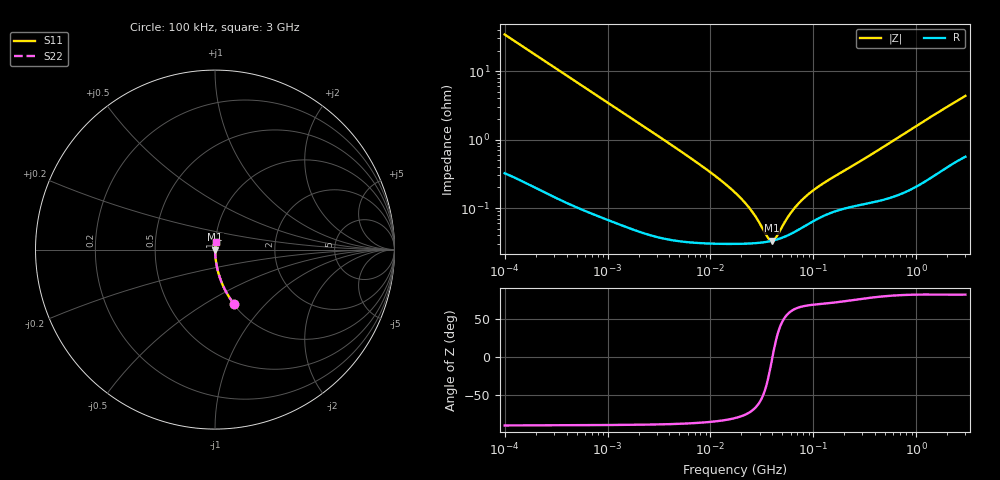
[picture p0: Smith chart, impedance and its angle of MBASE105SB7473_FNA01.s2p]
! MBASE105SB7473_FNA01  S-PARAMETER MODEL  ( Standard Model )
! Model Generated by TAIYO YUDEN Corporation (http://www.ty-top.com)
! Version 1.0
! TAIYO YUDEN Control No. 220601
! Copyright(c) 2013 TAIYO YUDEN CO.,LTD. All Rights Reserved.
! Product Description (link to TY-COMPAS)
! https://ds.yuden.co.jp/TYCOMPAS/or/detail?pn=MBASE105SB7473KFNA01&u=M
! Products Name : Multilayer Ceramic Capacitors
! Characteristics :
!  Capacitance : 0.047 [uF] , Rated Voltage : 16 [V] , TCC : X7R
!  Case Size : 1.0 x 0.5 / 0.039 x 0.02 [mm/inch] , Thickness : 0.5 / 0.02 [mm/inch]
!  (Conditions: Temperature = 25 [degC] , DC Bias Voltage = 0 [V])
! External Node Assignments :
!  1  o---| |---o  2
! GND o---------o GND
! Frequency Range : 100kHz  -  3GHz  [ 401 STEP ]
# MHZ S RI R 50
! Freq[MHz].  S11 Real  S11 Imag  S21 Real  S21 Imag  S12 Real  S12 Imag  S22 Real  S22 Imag
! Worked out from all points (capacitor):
!   401 points, 100 kHz to 3 GHz, reference 50 ohm
!   read as one part in series: C = 46.3 nF near 105.3 kHz
!   lowest |Z| = 33.3 mohm at 39.51 MHz (marker M1)
!   series resonance near 39.99 MHz, so ESL is about 340 pH
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0.1  0.1078 -0.3054  0.8922 0.3054  0.8922 0.3054  0.1078 -0.3054
0.147195  0.054 -0.2208  0.946 0.2208  0.946 0.2208  0.054 -0.2208
0.228123  0.0241 -0.1475  0.9759 0.1475  0.9759 0.1475  0.0241 -0.1475
0.562235  0.00474 -0.0614  0.9953 0.0614  0.9953 0.0614  0.00474 -0.0614
3.161081  0.000493 -0.0111  0.9995 0.0111  0.9995 0.0111  0.000493 -0.0111
9.574722  0.000316 -0.00348  0.9997 0.00348  0.9997 0.00348  0.000316 -0.00348
17.7727  0.000302 -0.0016  0.9997 0.0016  0.9997 0.0016  0.000302 -0.0016
24.21403  0.000304 -0.000929  0.9997 0.000929  0.9997 0.000929  0.000304 -0.000929
28.26337  0.000309 -0.000629  0.9997 0.000629  0.9997 0.000629  0.000309 -0.000629
35.64176  0.000322 -0.000205  0.9997 0.000205  0.9997 0.000205  0.000322 -0.000205
37.52708  0.000327 -0.000113  0.9997 0.000113  0.9997 0.000113  0.000327 -0.000113
39.51212  0.000332 -2.11e-05  0.9997 2.11e-05  0.9997 2.11e-05  0.000332 -2.11e-05
41.60216  0.000339 7.05e-05  0.9997 -7.05e-05  0.9997 -7.05e-05  0.000339 7.05e-05
43.80277  0.000346 0.000162  0.9997 -0.000162  0.9997 -0.000162  0.000346 0.000162
55.23785  0.000394 0.000578  0.9996 -0.000578  0.9996 -0.000578  0.000394 0.000578
66.15861  0.000451 0.00091  0.9995 -0.00091  0.9995 -0.00091  0.000451 0.00091
79.23846  0.000527 0.00125  0.9995 -0.00125  0.9995 -0.00125  0.000527 0.00125
97.38194  0.000633 0.00165  0.9994 -0.00165  0.9994 -0.00165  0.000633 0.00165
136.1397  0.000814 0.00236  0.9992 -0.00236  0.9992 -0.00236  0.000814 0.00236
547.5153  0.00147 0.00874  0.9985 -0.00874  0.9985 -0.00874  0.00147 0.00874
1575.075  0.00369 0.0239  0.9963 -0.0239  0.9963 -0.0239  0.00369 0.0239
3000  0.00742 0.0426  0.9926 -0.0426  0.9926 -0.0426  0.00742 0.0426
